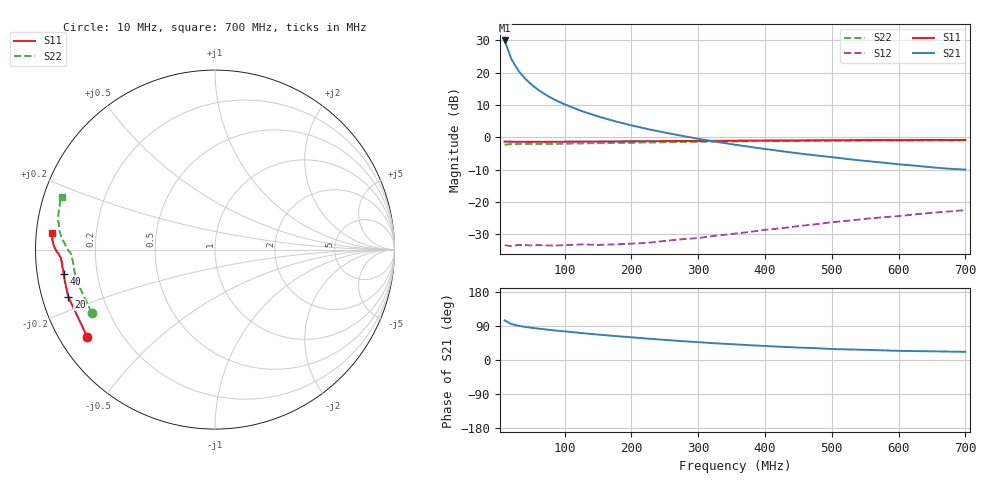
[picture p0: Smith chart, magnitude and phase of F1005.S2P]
! Date: Mon Aug 07 13:35:18 1995
# MHZ  S  MA  R  50.0000
!  POLYFET RF DEVICES
!  F1005
!  S PARAMETERS
!  VDS=28V, IDQ=800mA
!FREQ  S11MAG S11ANG S21MAG S21ANG S12MAG S12ANG S22MAG S22ANG
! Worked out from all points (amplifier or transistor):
!   34 points, 10 MHz to 700 MHz, reference 50 ohm
!   highest |S21| = 30.0 dB at 10 MHz (marker M1)
!   |S21| within 3 dB of that: start of sweep to 15.27 MHz
!   unconditionally stable (mu >= 1): 166.2 MHz to 535.7 MHz
!   at 60 MHz: K = 0.42, MSG = 24.0 dB, |S12| = -33.3 dB
!   at 300 MHz: K = 1.25, MAG = 12.3 dB, |S12| = -31.1 dB
!   at 700 MHz: K = 0.92, MSG = 6.3 dB, |S12| = -22.5 dB
!   S11 on the Smith chart (normalised r, x): 10 MHz: 0.08, -0.31; 20 MHz: 0.08, -0.16; 40 MHz: 0.08, -0.08; 700 MHz: 0.04, +0.05
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10  0.8622 -145.7  31.56 104.6  0.02157 17.1  0.7728 -152.9
20  0.8587 -162.1  16.39 94.9  0.0208 11.3  0.7864 -166.1
30  0.8548 -168.0  10.98 90.6  0.02169 10.2  0.7914 -170.8
40  0.8545 -170.8  8.234 87.5  0.02168 10.7  0.7939 -173.1
50  0.854 -172.6  6.581 85.1  0.02136 10.7  0.7933 -174.6
60  0.8571 -173.9  5.47 82.9  0.02162 12.6  0.7958 -175.9
70  0.8537 -174.6  4.672 80.8  0.02138 13.4  0.7981 -176.5
80  0.8569 -175.3  4.074 78.9  0.02131 12.6  0.7979 -177.1
90  0.8558 -175.7  3.613 77.1  0.02141 15.9  0.7991 -177.5
100  0.8592 -176.0  3.241 75.5  0.02158 16.2  0.7999 -177.9
125  0.8599 -176.9  2.565 71.1  0.02212 19.0  0.8077 -178.9
150  0.8625 -177.3  2.107 67.1  0.02175 23.3  0.8162 -179.5
175  0.8678 -177.8  1.781 63.4  0.02216 29.1  0.8211 179.7
200  0.8697 -178.2  1.536 59.9  0.02271 33.7  0.8279 179.0
225  0.8724 -178.6  1.341 56.3  0.02343 37.7  0.8348 178.2
250  0.8752 -178.8  1.188 53.0  0.02509 42.5  0.8397 177.5
300  0.8851 -179.5  0.9517 47.0  0.02778 50.6  0.8566 175.8
375  0.8908 179.7  0.7191 39.2  0.03437 57.7  0.8732 173.1
425  0.8959 178.9  0.6113 34.7  0.0394 60.6  0.8798 171.3
475  0.9003 178.2  0.5278 31.3  0.0453 62.7  0.889 169.4
600  0.9078 176.0  0.3841 24.2  0.06062 63.3  0.8988 164.7
700  0.9141 174.3  0.3176 21.6  0.07482 62.7  0.9022 161.1
